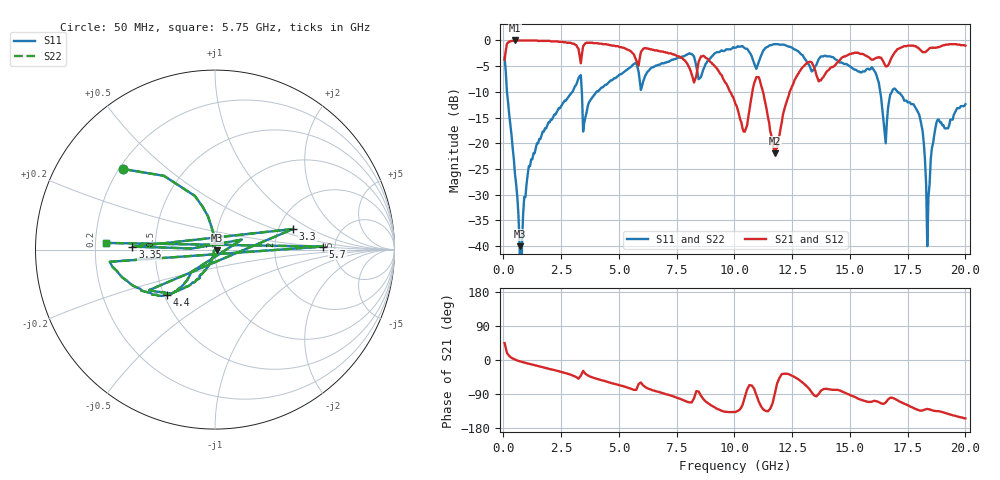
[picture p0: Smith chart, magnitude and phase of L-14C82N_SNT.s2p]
#	mhz	s	ma	r	50
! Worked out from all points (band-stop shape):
!   400 points, 50 MHz to 20 GHz, reference 50 ohm
!   highest |S21| = 0.00 dB at 500 MHz (marker M1); lowest = -21.9 dB at 11.75 GHz (marker M2)
!   |S21| within 3 dB of the highest: 71.89 MHz to 3.301 GHz (3.229 GHz wide, 191 % of centre); 16.85 GHz to end of sweep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
!   lowest |S11| = -40.0 dB at 700 MHz (marker M3), VSWR 1.02, Z = 50.9 - j0.437 ohm
!   |S11| at or under -10 dB: 152.4 MHz to 2.981 GHz (2.829 GHz wide, 181 % of centre); 3.394 GHz to 4.031 GHz (637.5 MHz wide, 17.2 % of centre); 17.07 GHz to end of sweep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
!   |S22| runs from - to -0.7 dB; largest |S21 - S12| = 0
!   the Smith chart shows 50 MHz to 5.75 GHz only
!   S11 on the Smith chart (normalised r, x): 50 MHz: 0.22, +0.36; 3.3 GHz: 2.40, +0.69; 3.35 GHz: 0.37, +0.02; 4.4 GHz: 0.51, -0.30; 5.7 GHz: 3.99, +0.21; 5.75 GHz: 0.24, +0.03
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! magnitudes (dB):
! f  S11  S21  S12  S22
! 50 MHz  -3.3  -3.7  -3.7  -3.3
! 500 MHz  -26.0  0.0  0.0  -26.0
! 700 MHz  -40.0  0.0  0.0  -40.0
! 750 MHz  -  0.0  0.0  -
! 800 MHz  -40.0  0.0  0.0  -40.0
! 1.1 GHz  -24.4  0.0  0.0  -24.4
! 3.3 GHz  -6.9  -3.0  -3.0  -6.9
! 3.35 GHz  -6.7  -4.4  -4.4  -6.7
! 3.4 GHz  -10.5  -2.6  -2.6  -10.5
! 4.4 GHz  -8.6  -0.7  -0.7  -8.6
! 5.7 GHz  -4.4  -3.3  -3.3  -4.4
! 5.75 GHz  -4.3  -3.9  -3.9  -4.3
! 6.7 GHz  -4.7  -2.0  -2.0  -4.7
! 10.05 GHz  -1.4  -12.4  -12.4  -1.4
! 11.05 GHz  -4.3  -7.1  -7.1  -4.3
! 11.75 GHz  -0.7  -21.9  -21.9  -0.7
! 13.35 GHz  -6.0  -4.3  -4.3  -6.0
! 16.7 GHz  -11.7  -4.4  -4.4  -11.7
! 18 GHz  -14.4  -1.6  -1.6  -14.4
! 18.35 GHz  -40.0  -1.9  -1.9  -40.0
! 18.75 GHz  -15.9  -1.4  -1.4  -15.9
! 20 GHz  -12.4  -1.0  -1.0  -12.4
